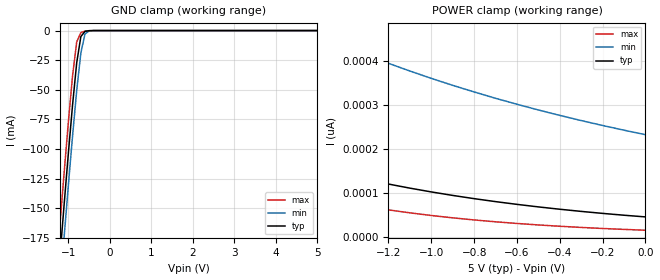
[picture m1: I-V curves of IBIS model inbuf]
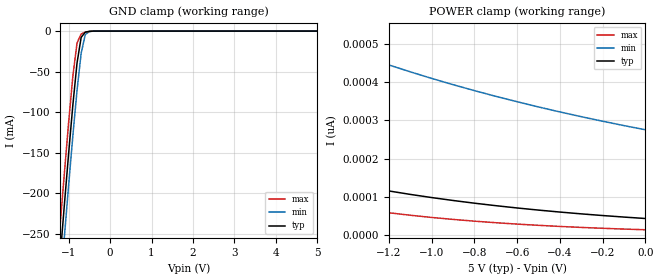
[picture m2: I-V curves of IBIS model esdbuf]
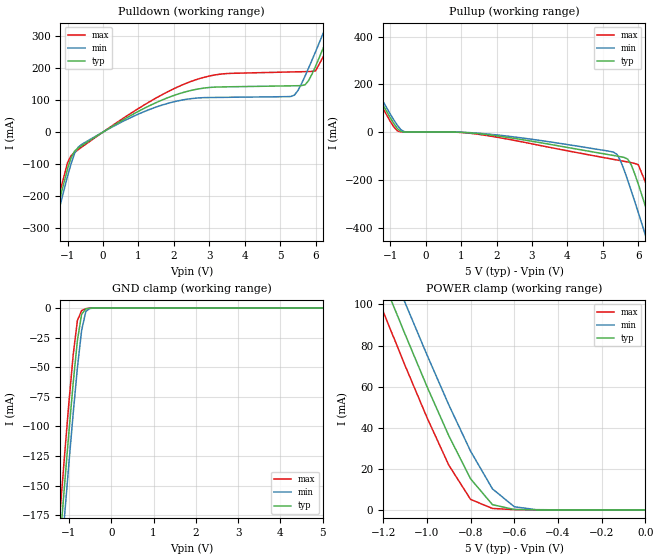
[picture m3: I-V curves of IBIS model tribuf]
|   * 62374L.ibs * IBIS 1.1 Model for FCT162374T/AT/CT/ET
[IBIS Ver]	1.1
[Comment char]	|_char
[File name]	74fct162374t.ibs
[Date]		Mon Nov 25 18:23:31 1996
[File Rev]	1.0
[Source] s2ibis Version 1.3 SPICE to IBIS converter
   Integrated Device Technology, Inc.
[Notes]
... Temperatures: typ=50C, min=0C, max=100C
... Ramp rate based on 500 ohm load
... User should use package parameters of their own applications.
... Copyright 1996 IIntegrated Device Technology, Inc.
[Disclaimer] IDT provides this model for simulation purpose only.
|   IDT reserves the right to modify this IBIS model in
|   the event of product upgrades applicable to this
|   particular product.
|   COMPONENT: FCT162374T/AT/CT/ET
[Component]	FCT162374T/AT/CT/ET
[Manufacturer]	Integrated Device Technology Inc.
[Package]
| SO48-1 SSOP
| variable   typ   min   max
R_pkg   10m   9m   11m
L_pkg   3.5nh   3.0nh   4.0nh
C_pkg   0.3pf   0.26pf   0.34pf
[Pin]  signal_name   model_name   R_pin  L_pin  C_pin
1   1OEb   inbuf
2   1O1   tribuf
3   1O2   tribuf
4   GND   GND
5   1O3   tribuf
6   1O4   tribuf
7   VCC   POWER
8   1O5   tribuf
9   1O6   tribuf
10   GND   GND
11   1O7   tribuf
12   1O8   tribuf
13   2O1   tribuf
14   2O2   tribuf
15   GND   GND
16   2O3   tribuf
17   2O4   tribuf
18   VCC   POWER
19   2O5   tribuf
20   2O6   tribuf
21   GND   GND
22   2O7   tribuf
23   2O8   tribuf
24   2OEb   inbuf
25   2CLK   inbuf
26   2D8   esdbuf
27   2D7   esdbuf
28   GND   GND
29   2D6   esdbuf
30   2D5   esdbuf
31   VCC   POWER
32   2D4   esdbuf
33   2D3   esdbuf
34   GND   GND
35   2D2   esdbuf
36   2D1   esdbuf
37   1D8   esdbuf
38   1D7   esdbuf
39   GND   GND
40   1D6   esdbuf
41   1D5   esdbuf
42   VCC   POWER
43   1D4   esdbuf
44   1D3   esdbuf
45   GND   GND
46   1D2   esdbuf
47   1D1   esdbuf
48   1CLK   inbuf
| Models and submodels in the file (3): inbuf (Input), esdbuf (Input), tribuf (3-state)
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|   MODEL inbuf
[Model]		inbuf
Model_type	Input
C_comp   5.0pF   5.0pF   5.0pF
[Voltage range]   5.000   4.750   5.250
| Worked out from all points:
|   GND clamp passes 1 mA (typ) near -0.61 V on its own axis
[GND_clamp]
|  Voltage   I(typ)   I(min)   I(max)
-5V       -1.941A    -1.966A    -1.918A
-1.3V     -232.8mA   -260.1mA   -205.9mA
-1.2V     -188.6mA   -215.9mA   -161.7mA
-1.1V     -145.1mA   -172.4mA   -118.3mA
-1V       -102.8mA   -129.8mA   -76.45mA
-900mV    -62.51mA   -88.66mA   -37.88mA
-800mV    -27.03mA   -50.37mA   -9.521mA
-700mV    -5.009mA   -18.75mA   -1.725mA
-600mV    -627.2uA   -2.79mA    -425.3uA
-500mV    -121uA     -293.6uA   -54.36uA
5V        45.25pA    258.7pA    11.12pA
[POWER_clamp]
|  Voltage   I(typ)   I(min)   I(max)
-5V       2.423nA    2.665nA    4.499nA
-3V       506.5pA    937.5pA    483.4pA
-2.9V     467.9pA    891.5pA    431.6pA
-2.7V     399.2pA    806.8pA    343.9pA
-2.5V     340.5pA    730.9pA    273.8pA
-2.2V     268pA      631.4pA    194.3pA
-1.9V     210.8pA    546.8pA    137.7pA
-1.6V     165.7pA    474.7pA    97.38pA
-1.2V     120pA      394.6pA    61.22pA
-800mV    86.8pA     329.5pA    38.38pA
-400mV    62.71pA    276.2pA    24pA
0V        45.25pA    232.3pA    14.96pA
|   MODEL esdbuf
[Model]		esdbuf
Model_type	Input
C_comp   5.0pF   5.0pF   5.0pF
[Voltage range]   5.000   4.750   5.250
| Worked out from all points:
|   GND clamp passes 1 mA (typ) near -0.57 V on its own axis
[GND_clamp]
|  Voltage   I(typ)   I(min)   I(max)
-5V       -2.822A    -2.858A    -2.787A
-1.3V     -338.5mA   -378.1mA   -299.4mA
-1.2V     -274.3mA   -314mA     -235.2mA
-1.1V     -211.1mA   -250.7mA   -172.2mA
-1V       -149.6mA   -188.8mA   -111.4mA
-900mV    -91.07mA   -129mA     -55.48mA
-800mV    -39.59mA   -73.39mA   -14.74mA
-700mV    -7.773mA   -27.46mA   -3.57mA
-600mV    -1.309mA   -4.281mA   -1.305mA
-500mV    -357uA     -550.8uA   -359.4uA
-400mV    -25.95uA   -39.88uA   -25.63uA
5V        43.93pA    303.8pA    10.83pA
[POWER_clamp]
|  Voltage   I(typ)   I(min)   I(max)
-5V       2.327nA    2.668nA    4.315nA
-3.2V     570.4pA    1.085nA    581.2pA
-3.1V     527.2pA    1.034nA    519.1pA
-2.9V     450.1pA    941.5pA    414pA
-2.6V     354.8pA    819.3pA    294.4pA
-2.3V     279.5pA    715pA      209.1pA
-2V       220.1pA    625.8pA    148.3pA
-1.6V     159.8pA    526.4pA    93.59pA
-1.3V     125.6pA    463.8pA    66.16pA
-900mV    91.01pA    393.5pA    41.58pA
-500mV    65.88pA    335.2pA    26.08pA
0V        43.93pA    275.6pA    14.52pA
|   MODEL tribuf
[Model]		tribuf
Model_type	3-state
Polarity	Non-Inverting
Enable		Active-High
C_comp   5.0pF   5.0pF   5.0pF
[Voltage range]   5.000   4.750   5.250
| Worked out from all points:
|   slope of the pulldown table from 0 to 0.75 V, typ, clamps not added: 15.1 ohm
|   slope of the pullup table from 0 to 0.75 V, typ, clamps not added: 8.43 kohm
|   GND clamp passes 1 mA (typ) near -0.61 V on its own axis
|   POWER clamp passes 1 mA (typ) near -0.64 V on its own axis
[Pulldown]
|  Voltage   I(typ)   I(min)   I(max)
-5V       -2.038A    -2.045A    -2.035A
-1.8V     -474.6mA   -497.4mA   -454.3mA
-1.4V     -287.8mA   -312.3mA   -265mA
-1V       -114.2mA   -137.5mA   -95.61mA
-700mV    -49.72mA   -47.12mA   -54.88mA
2.4V      127.6mA    103mA      154.4mA
5.4V      144.4mA    115.2mA    187.8mA
5.8V      160.2mA    199.4mA    188.8mA
6V        205.6mA    251.3mA    191mA
6.4V      310.9mA    358.4mA    273.5mA
6.8V      420.1mA    467.3mA    382.4mA
10V       1.313A     1.353A     1.285A
[GND_clamp]
|  Voltage   I(typ)   I(min)   I(max)
-5V       -2.037A    -2.045A    -2.035A
-1.3V     -238.4mA   -263.9mA   -214.4mA
-1.2V     -192.9mA   -218.8mA   -168.4mA
-1.1V     -148.2mA   -174.4mA   -123.3mA
-1V       -104.8mA   -131.1mA   -79.86mA
-900mV    -63.7mA    -89.37mA   -40mA
-800mV    -27.59mA   -50.71mA   -10.6mA
-700mV    -5.192mA   -18.87mA   -2.12mA
-600mV    -668.6uA   -2.818mA   -511.9uA
-500mV    -124.7uA   -296uA     -63.3uA
5V        43.73pA    43.51nA    10.75pA
[Pullup]
|  Voltage   I(typ)   I(min)   I(max)
-5V       1.162A     1.168A     1.158A
-2.6V     493.9mA    505.4mA    483mA
-2.2V     383.3mA    395.8mA    371.3mA
-900mV    36.14mA    51.19mA    21.81mA
-600mV    161.7uA    1.51mA     127.8uA
1.4V      -5.345mA   -3.804mA   -7.675mA
5.3V      -98.09mA   -84.06mA   -114.4mA
5.8V      -137.8mA   -246.1mA   -128.1mA
6V        -218.7mA   -337.8mA   -136.9mA
6.4V      -403.3mA   -526.6mA   -283.8mA
6.8V      -594.4mA   -718.3mA   -472.9mA
10V       -2.155A    -2.275A    -2.037A
[POWER_clamp]
|  Voltage   I(typ)   I(min)   I(max)
-5V       1.162A     1.168A     1.158A
-1.3V     138.1mA    153mA      123.3mA
-1.2V     111.6mA    126.8mA    96.57mA
-1.1V     85.56mA    100.9mA    70.32mA
-1V       60.16mA    75.57mA    45.06mA
-900mV    36.14mA    51.19mA    21.81mA
-800mV    15.1mA     28.57mA    5.098mA
-700mV    2.54mA     10.23mA    668.6uA
-600mV    161.7uA    1.51mA     127.8uA
-500mV    7.595uA    97.93uA    10.32uA
0V        43.73pA    228.5pA    14.47pA
[Ramp]
|  variable   typ   min   max
dV/dt_r   2.09/0.41n   1.88/0.54n   2.31/0.31n
dV/dt_f   2.91/0.52n   2.76/0.73n   3.07/0.37n
